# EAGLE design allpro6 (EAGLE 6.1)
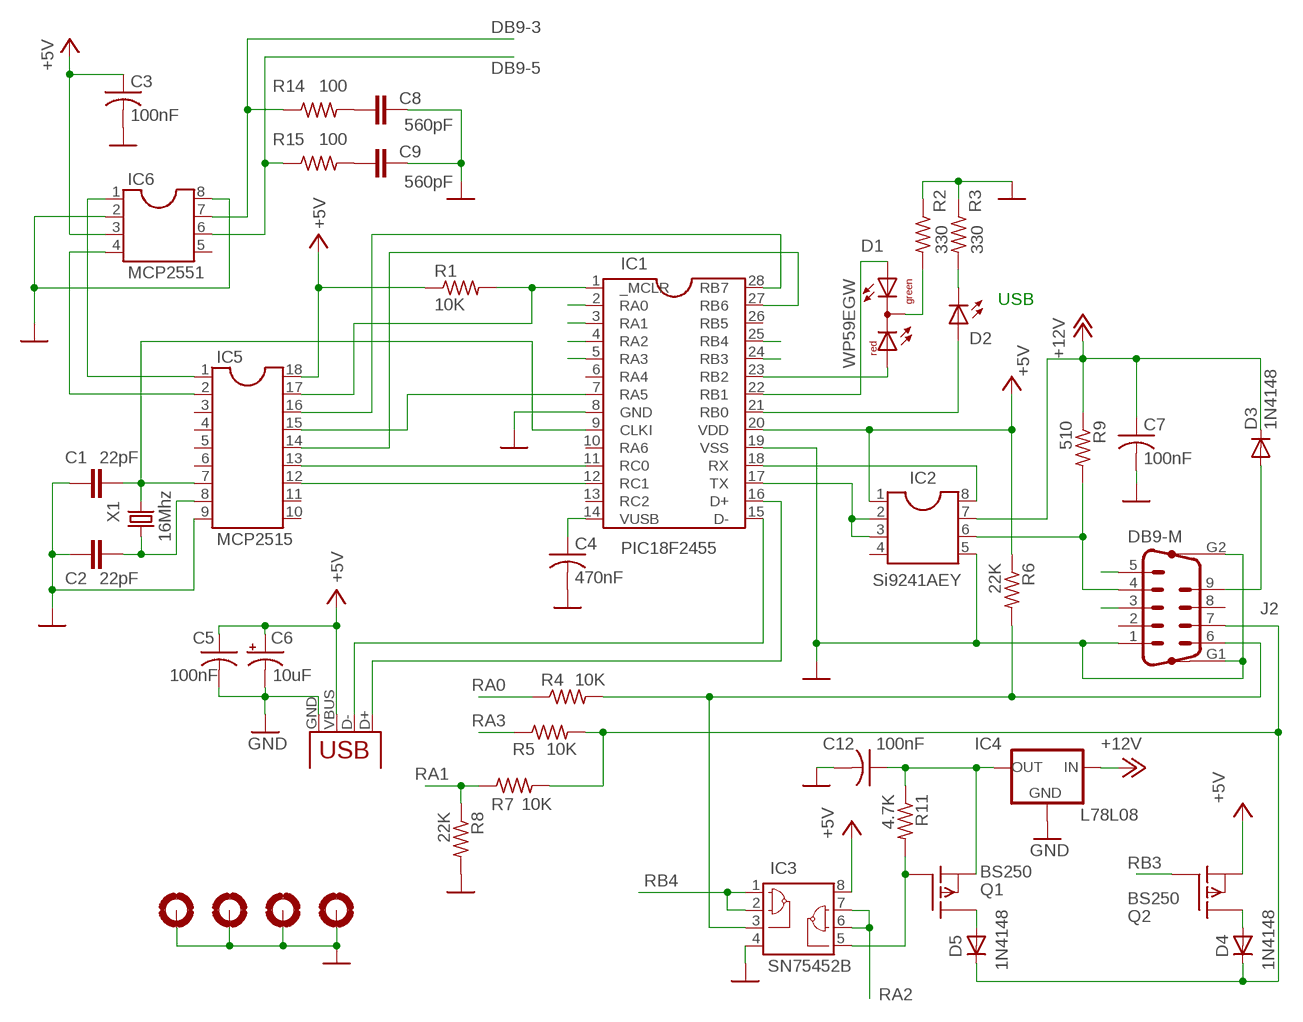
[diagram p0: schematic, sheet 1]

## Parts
C1  22pF  C2.5/2  [C2.5-2]
C2  22pF  C2.5/2  [C2.5-2]
C3  100nF  C-US050-025X075  [C050-025X075]
C4  470nF  C-US050-035X075  [C050-035X075]
C5  100nF  C-US050-025X075  [C050-025X075]
C6  10uF  CPOL-USE2-4  [E2-4]
C7  100nF  C-US050-025X075  [C050-025X075]
C8  560pF  C2.5/2  [C2.5-2]
C9  560pF  C2.5/2  [C2.5-2]
C12  100nF  C-US050-025X075  [C050-025X075]
D1  WP59EGW  DUOLED-RG-C  [DUOLED-C-5MM]
D2  LED5MM  [LED5MM]
D3  1N4148  1N4148M  [D035-10M]
D4  1N4148  1N4148M  [D035-10M]
D5  1N4148  1N4148M  [D035-10M]
H1  MOUNT-PAD-ROUND2.8  [2,8-PAD]
H2  MOUNT-PAD-ROUND2.8  [2,8-PAD]
H3  MOUNT-PAD-ROUND2.8  [2,8-PAD]
H4  MOUNT-PAD-ROUND2.8  [2,8-PAD]
IC1  PIC18F2455  PIC18F2455-EC  [DIL28]
IC2  Si9241AEY  SO-8  [SO-8]
IC3  SN75452B  [DIL08]
IC4  L78L08  78LXX  [78LXX]
IC5  MCP2515  DIL18  [DIL18]
IC6  MCP2551  DIL8  [DIL08]
J1  USB-B-H  [USB-B-H]
J2  DB9-M  M09HP  [M09HP]
Q1  BS250  [TO92]
Q2  BS250  [TO92]
R1  10K  R-US_0207/10  [0207/10]
R2  330  R-US_0207/10  [0207/10]
R3  330  R-US_0207/10  [0207/10]
R4  10K  R-US_0207/10  [0207/10]
R5  10K  R-US_0207/10  [0207/10]
R6  22K  R-US_0207/10  [0207/10]
R7  10K  R-US_0207/10  [0207/10]
R8  22K  R-US_0207/10  [0207/10]
R9  510  R-US_0207/10  [0207/10]
R11  4.7K  R-US_0207/10  [0207/10]
R14  100  R-US_0207/10  [0207/10]
R15  100  R-US_0207/10  [0207/10]
X1  16Mhz  CRYTALHC49S  [HC49/S]

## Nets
+5V: C3.1 C5.1 C6.+ IC1.20(VDD) IC2.1 IC3.8 IC5.18 IC6.3 J1.VBUS Q2.1(S) R1.1 R6.1
+12V: C7.1 D3.C IC2.7 IC4.IN R9.1
DB9-3: IC6.7 J2.3 R14.1
DB9-5: IC6.6 J2.5 R15.1
GND: C1.1 C2.2 C3.2 C4.2 C5.2 C6.- C7.2 C8.1 C9.1 C12.2 H1.B2,8(MOUNT) H2.B2,8(MOUNT) H3.B2,8(MOUNT) H4.B2,8(MOUNT) IC1.8(GND) IC1.19(VSS) IC2.5 IC3.4 IC4.GND IC5.9 IC6.2 IC6.8 J1.GND J2.1 J2.G1 J2.G2 R2.1 R3.1 R8.2
N$1: IC3.3 J2.6 R4.2 R6.2
N$3: D1.AR IC1.23(RB2)
N$4: IC5.2 IC6.4
N$5: D2.A IC1.21(RB0)
N$6: IC2.6 J2.4 R9.2
N$7: D3.A J2.9
N$8: D1.C R2.2
N$10: D2.K(C) R3.2
N$11: IC1.15(D-) J1.D-
N$12: IC1.16(D+) J1.D+
N$14: D1.AX(AG) IC1.22(RB1)
N$15: IC1.27(RB6) IC5.14
N$16: IC1.28(RB7) IC5.16
N$17: IC1.1(_MCLR) IC5.17 R1.2
N$18: D4.C D5.C J2.7 R5.2 R7.2
N$19: IC5.1 IC6.1
N$21: IC1.17(TX) IC2.2 IC2.3
N$22: C4.1 IC1.14(VUSB)
N$23: IC1.18(RX) IC2.8
N$25: D4.A Q2.3(D)
N$28: IC3.5 Q1.2(G) R11.2
N$35: C9.2 R15.2
N$36: C8.2 R14.2
N$37: IC1.7(RA5) IC5.15
N$40: C1.2 IC1.9(CLKI) IC5.7 X1.2
N$41: C2.1 IC5.8 X1.1
N$43: D5.A Q1.3(D)
N$45: C12.1 IC4.OUT Q1.1(S) R11.1
RA0: IC1.2(RA0) R4.1
RA1: IC1.3(RA1) R7.1 R8.1
RA2: IC1.4(RA2) IC3.6 IC3.7
RA3: IC1.5(RA3) R5.1
RB3: IC1.24(RB3) Q2.2(G)
RB4: IC1.25(RB4) IC3.1 IC3.2
RC0: IC1.11(RC0) IC5.13
RC1: IC1.12(RC1) IC5.12
Unconnected: IC1.6(RA4) IC1.10(RA6) IC1.13(RC2) IC1.26(RB5) IC2.4 IC5.3 IC5.4 IC5.5 IC5.6 IC5.10 IC5.11 IC6.5 J2.2 J2.8

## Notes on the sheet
- USB

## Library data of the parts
C1 C2 C8 C9 = capacitor-wima:C: CAPACITOR
C3-C5 C7 C12 = rcl:C-US: CAPACITOR, American symbol
C6 = rcl:CPOL-US: POLARIZED CAPACITOR, American symbol
D1 = led:DUOLED-RG-C: DUO LED 2 colors (red/green), 5 mm, round, common Cathode www.ligitek.com or other producers.
D2 = led:LED: LED
D3-D5 = diode:1N4148: DIODE
H1-H4 = holes:MOUNT-PAD-ROUND: MOUNTING PAD, round
IC1 = pic18f2455:PIC18F2455-EC
IC2 = so-8:SO-8
IC3 = 7545x:SN75452B
IC4 = v-reg:78LXX: VOLTAGE REGULATOR
IC5 = ic-package:DIL18: Dual In Line
IC6 = ic-package:DIL8: Dual In Line / Socket
J1 = con-usb:USB: USB Connectors
J2 = con-subd:M09HP: SUB-D; OC_FARNELL: unknown; OC_NEWARK: unknown
Q1 Q2 = transistor-fet:BS250: P-Channel Enhancement MOSFET -20V; -2A; 2,0Ohm
R1-R9 R11 R14 R15 = rcl:R-US_: RESISTOR, American symbol
X1 = crystal:CRYTAL: CRYSTAL

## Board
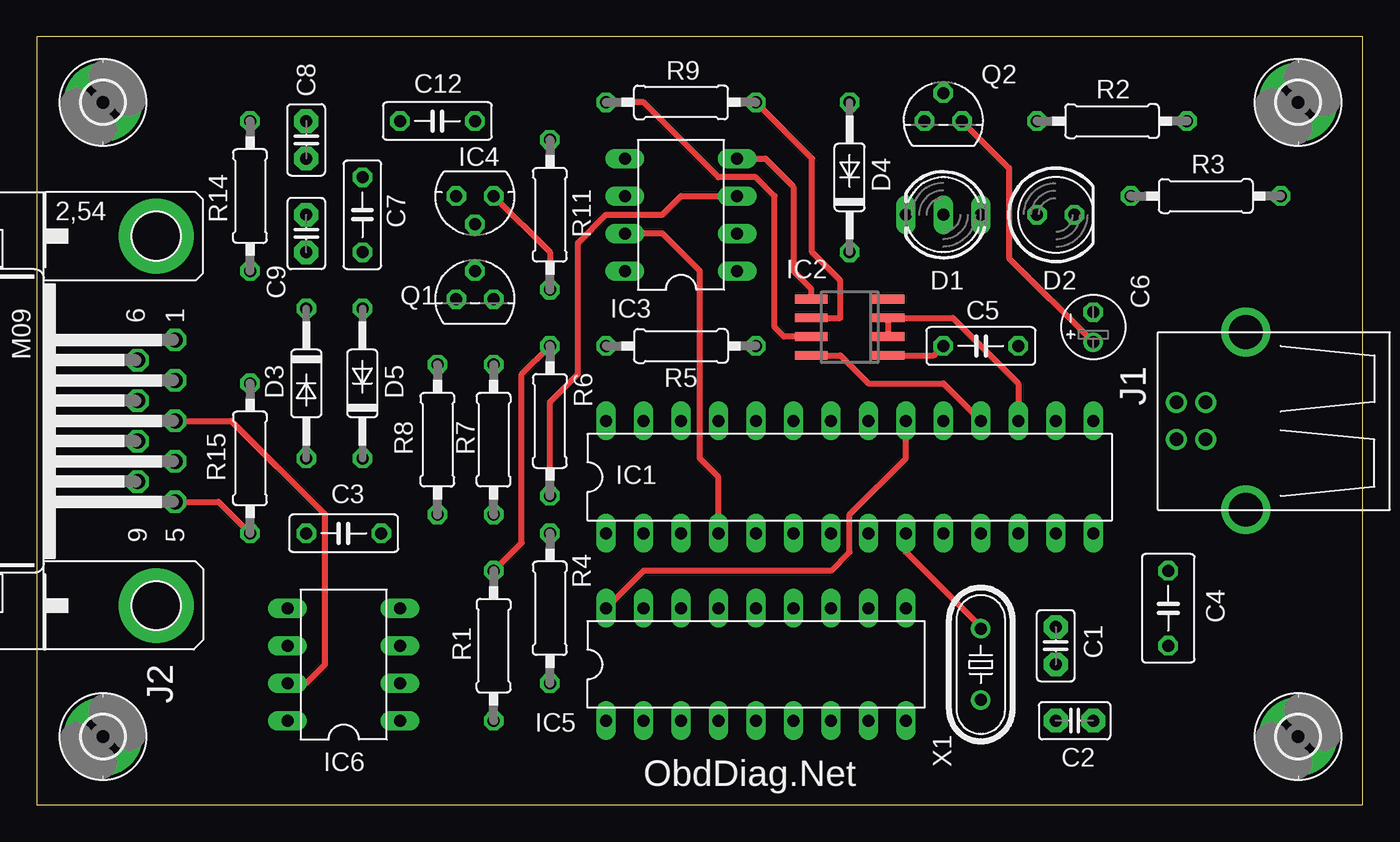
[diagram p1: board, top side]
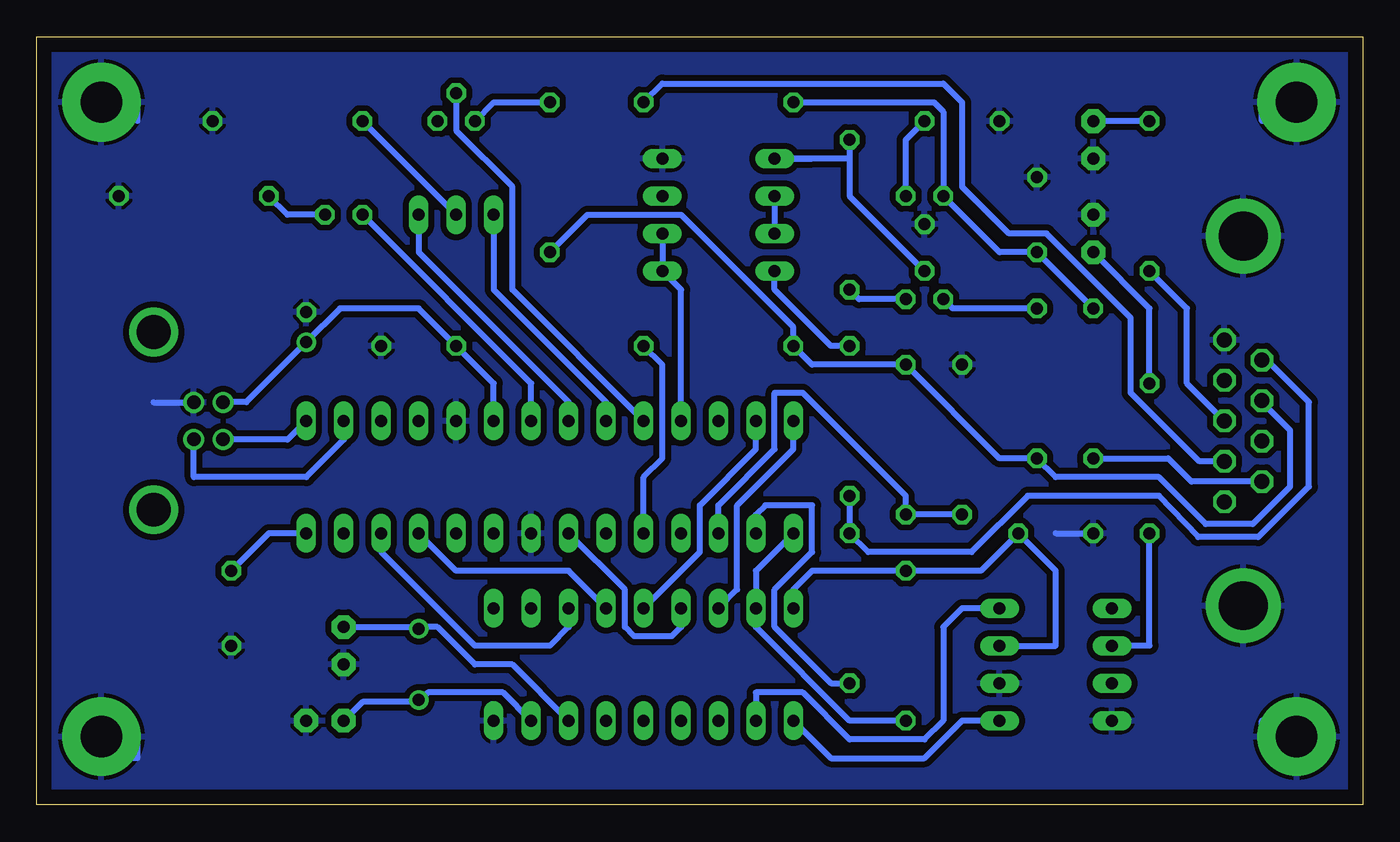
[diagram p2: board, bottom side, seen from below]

Size 89.84 x 52.06 mm. Coordinates in mm from the lower left corner, seen from the top.
Outline: 0,0 89.84,0 89.84,52.06 0,52.06 0,0
Copper layers (1*16): Top 0.035mm / dielectric 1.5mm / Bottom 0.035mm
Design rules: minimum track width 10mil, minimum drill 24mil, track to track 8mil, track to pad 8mil, pad to pad 8mil, via to via 8mil, smd to smd 8mil, copper to edge 40mil, drill to drill 8mil, minimum pad ring 10mil, minimum via ring 8mil, stop-mask expansion 4mil, vias tented up to drill 0mil, thermal gap 10mil

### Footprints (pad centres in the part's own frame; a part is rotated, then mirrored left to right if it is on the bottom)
C2.5-2 = drill 0.813 pad 1.6 octagon: 1 -1.27,0; 2 1.27,0
C050-025X075 = drill 0.813 octagon: 1 -2.54,0; 2 2.54,0
C050-035X075 = drill 0.813 octagon: 1 -2.54,0; 2 2.54,0
E2-4 = drill 0.813 pad 1.27: + -1.016,0 | drill 0.813 pad 1.27 octagon: - 1.016,0
DUOLED-C-5MM = drill 0.813 long: AR 2.54,0; AX -2.54,0; C 0,0
LED5MM = drill 0.813 octagon: A -1.27,0; K 1.27,0
D035-10M = drill 0.813 octagon: A 5.08,0; C -5.08,0
2,8-PAD = drill 2.8 pad 5.334: B2,8 0,0
DIL28 = drill 0.813 long: 1 -16.51,-3.81; 2 -13.97,-3.81; 3 -11.43,-3.81; 4 -8.89,-3.81; 5 -6.35,-3.81; 6 -3.81,-3.81; 7 -1.27,-3.81; 8 1.27,-3.81; 9 3.81,-3.81; 10 6.35,-3.81; 11 8.89,-3.81; 12 11.43,-3.81; 13 13.97,-3.81; 14 16.51,-3.81; 15 16.51,3.81; 16 13.97,3.81; 17 11.43,3.81; 18 8.89,3.81; 19 6.35,3.81; 20 3.81,3.81; 21 1.27,3.81; 22 -1.27,3.81; 23 -3.81,3.81; 24 -6.35,3.81; 25 -8.89,3.81; 26 -11.43,3.81; 27 -13.97,3.81; 28 -16.51,3.81
SO-8 = smd 0.6 x 2.2: 1 -1.905,-2.6; 2 -0.635,-2.6; 3 0.635,-2.6; 4 1.905,-2.6; 5 1.905,2.6; 6 0.635,2.6; 7 -0.635,2.6; 8 -1.905,2.6
DIL08 = drill 0.813 long: 1 -3.81,-3.81; 2 -1.27,-3.81; 3 1.27,-3.81; 4 3.81,-3.81; 5 3.81,3.81; 6 1.27,3.81; 7 -1.27,3.81; 8 -3.81,3.81
78LXX = drill 0.813 octagon: GND 0,1.905; IN 1.27,0; OUT -1.27,0
DIL18 = drill 0.813 long: 1 -10.16,-3.81; 2 -7.62,-3.81; 3 -5.08,-3.81; 4 -2.54,-3.81; 5 0,-3.81; 6 2.54,-3.81; 7 5.08,-3.81; 8 7.62,-3.81; 9 10.16,-3.81; 10 10.16,3.81; 11 7.62,3.81; 12 5.08,3.81; 13 2.54,3.81; 14 0,3.81; 15 -2.54,3.81; 16 -5.08,3.81; 17 -7.62,3.81; 18 -10.16,3.81
USB-B-H = drill 0.914: D+ 0,1.25; D- 1.981,1.25; GND 0,-1.25; VBUS 1.981,-1.25 | drill 2.286: P$1 -2.718,-6.02; P$2 -2.718,6.02
M09HP = drill 1.016 octagon: 1 -5.486,1.27; 2 -2.743,1.27; 3 0,1.27; 4 2.743,1.27; 5 5.486,1.27; 6 -4.115,-1.27; 7 -1.372,-1.27; 8 1.372,-1.27; 9 4.115,-1.27 | drill 3.302 pad 5.08: G1 -12.522,0; G2 12.522,0
TO92 = drill 0.813 octagon: 1 1.27,0; 2 0,1.905; 3 -1.27,0
0207/10 = drill 0.813 octagon: 1 -5.08,0; 2 5.08,0
HC49/S = drill 0.813: 1 -2.413,0; 2 2.413,0

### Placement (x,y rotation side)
C1  69.05,10.79 90 top
C2  70.32,5.71 0 top
C3  20.79,18.41 180 top
C4  76.67,13.33 270 top
C5  63.97,31.11 0 top
C6  71.59,32.38 90 top
C7  22.06,40 90 top
C8  18.25,45.08 90 top
C9  18.25,38.73 270 top
C12  27.14,46.35 180 top
D1  61.43,40 180 top
D2  69.05,40 0 top
D3  18.25,28.57 270 top
D4  55.08,42.54 90 top
D5  22.06,28.57 90 top
H1  4.47,4.63 0 top
H2  4.47,47.63 0 top
H3  85.47,4.63 0 top
H4  85.47,47.63 0 top
IC1  55.08,22.22 0 top
IC2  55.08,32.38 90 top
IC3  43.65,40 90 top
IC4  29.68,41.27 180 top
IC5  48.73,9.52 0 top
IC6  20.79,9.52 90 top
J1  79.21,26.03 180 top
J2  8.09,26.03 270 top
Q1  29.68,34.29 0 top
Q2  61.43,46.35 0 top
R1  30.95,10.79 270 top
R2  72.86,46.35 180 top
R3  79.21,41.27 180 top
R4  34.76,13.33 90 top
R5  43.65,31.11 180 top
R6  34.76,26.03 270 top
R7  30.95,24.76 90 top
R8  27.14,24.76 90 top
R9  43.65,47.62 0 top
R11  34.76,40 90 top
R14  14.44,41.27 90 top
R15  14.44,23.49 90 top
X1  63.97,9.52 90 top

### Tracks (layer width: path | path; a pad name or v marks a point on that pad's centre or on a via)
+5V
  Top 0.406: IC2.1 60.8,30.47 C5.1 | R1.1 32.85,17.77 32.85,29.2 R6.1 | Q2.1 65.88,43.18 65.88,37.08 C6.+ | IC5.18 41.11,15.87 53.81,15.87 55.08,17.14 55.08,19.68 58.89,23.49 IC1.20
  Bottom 0.406: J1.VBUS 76.69,27.28 76.67,27.3 75.65,27.3 C6.+ 69.3,33.65 63.97,33.65 C5.1 58.89,28.57 IC1.20 | IC6.3 20.79,10.79 20.79,15.87 C3.1 25.87,15.87 R1.1 37.3,15.87 38.57,14.6 IC5.18 | R6.1 36.03,31.11 39.84,34.92 IC3.8
+12V
  Top 0.406: IC2.7 50.63,31.74 50,32.38 50,41.27 48.73,42.54 46.19,42.54 41.11,47.62 R9.1
  Bottom 0.406: D3.C C7.1 24.6,37.46 IC4.IN 28.41,46.98 29.04,47.62 R9.1
DB9-3
  Top 0.406: IC6.7 18.25,8.25 19.52,9.52 19.52,19.68 13.17,26.03 J2.3
  Bottom 0.406: J2.3 11.9,28.57 11.9,33.65 R14.1
DB9-5
  Top 0.406: J2.5 12.31,20.54 R15.1
  Bottom 0.406: R15.1 14.44,10.79 IC6.6
GND
  Top 0.406: IC3.4 49.37,43.81 51.27,41.91 51.27,36.19 52.48,34.98 IC2.5
  Bottom 0.406: 20.79,18.41 C3.2 | 81.94,27.28 J1.GND | 6.57,47.62 6.82,47.62 6.82,46.35 | 6.82,4.44 6.82,5.71 | 83.02,46.35 83.02,47.62 | 83.02,4.44 83.02,3.17 85.56,3.17
  pour Bottom (isolate 0.406): 0.47,51.43 89.37,51.43 89.37,0.63 0.47,0.63
N$1
  Top 0.406: R6.2 34.76,27.3 36.66,29.2 36.66,38.1 38.57,40 42.38,40 43.65,41.27 IC3.3
  Bottom 0.406: R6.2 R4.2 33.49,17.14 26.5,17.14 22.7,20.95 13.81,20.95 11.14,18.16 7.07,18.16 3.64,21.58 3.64,27.3 6.49,30.14 J2.6
N$3
  Bottom 0.406: IC1.23 51.27,27.3 58.89,34.92 D1.AR
N$4
  Bottom 0.406: IC5.2 41.11,7.62 37.94,7.62 34.76,4.44 29.68,4.44 28.41,5.71 28.41,12.06 27.14,13.33 IC6.4
N$5
  Bottom 0.406: IC1.21 56.35,28.57 D2.A
N$6
  Top 0.406: IC2.6 54.45,33.02 54.45,35.55 52.54,37.46 52.54,43.81 R9.2
  Bottom 0.406: J2.4 11.06,23.29 15.71,27.93 15.71,33.02 21.42,38.73 23.96,38.73 27.14,41.91 27.14,47.62 28.41,48.89 47.46,48.89 R9.2
N$7
  Bottom 0.406: D3.A 13.17,23.49 11.6,21.91 J2.9
N$8
  Bottom 0.406: D1.C R2.2
N$10
  Bottom 0.406: D2.K 72.86,40 R3.2
N$11
  Bottom 0.406: IC1.15 72.86,24.76 77.21,24.76 J1.D-
N$12
  Bottom 0.406: J1.D+ 79.21,22.22 71.59,22.22 69.05,24.76 IC1.16
N$14
  Bottom 0.406: IC1.22 53.81,27.3 63.97,37.46 D1.AX
N$15
  Bottom 0.406: IC1.27 41.11,24.12 44.92,20.31 44.92,17.14 IC5.14
N$16
  Bottom 0.406: IC1.28 38.57,24.12 42.38,20.31 42.38,14.6 IC5.16
N$17
  Bottom 0.406: R1.2 34.76,5.71 41.11,12.06 IC5.17 41.11,15.87 IC1.1
N$18
  Bottom 0.406: D4.C 52.54,40 46.19,40 38.57,32.38 R5.2 37.3,29.84 R7.2 24.6,23.49 D5.C 20.79,22.22 13.81,22.22 10.63,19.04 7.46,19.04 4.92,21.58 4.92,25.39 6.82,27.3 J2.7
N$19
  Bottom 0.406: IC6.1 27.14,5.71 29.68,3.17 36.03,3.17 IC5.1
N$21
  Top 0.406: IC2.2 IC2.3 62.06,33.02 66.51,28.57 IC1.17
N$22
  Bottom 0.406: C4.1 74.13,18.41 IC1.14
N$23
  Top 0.406: IC1.18 61.43,28.57 56.35,28.57 54.45,30.47 IC2.8
N$25
  Bottom 0.406: Q2.3 58.89,47.62 D4.A
N$28
  Bottom 0.406: 37.3,43.81 IC3.5 34.76,43.81 | Q1.2 34.76,41.27 34.76,43.81 | R11.2 34.76,43.81
N$35
  Bottom 0.406: C9.2 14.44,33.65 R15.2
N$36
  Bottom 0.406: R14.2 C8.2
N$37
  Bottom 0.406: IC1.7 50,14.6 50,12.06 49.37,11.43 46.82,11.43 46.19,12.06 IC5.15
N$40
  Top 0.406: IC1.9 58.89,17.14 63.97,12.06 X1.2
  Bottom 0.406: 64.1,12.06 X1.2 | IC5.7 57.62,9.52 60.16,9.52 62.7,12.06 63.97,12.06 64.1,12.06 | C1.2 64.1,12.06
N$41
  Bottom 0.406: 63.97,6.98 X1.1 | 63.97,6.98 67.78,6.98 C2.1 | IC5.8 58.25,7.62 63.34,7.62 63.97,6.98
N$43
  Bottom 0.406: D5.A 27.77,33.65 Q1.3
N$45
  Top 0.406: IC4.OUT 34.76,37.46 R11.1
  Bottom 0.406: IC4.OUT 30.95,45.08 C12.1 | Q1.1 34.12,34.29 R11.1
RA0
  Bottom 0.406: IC1.2 41.11,19.68 40.48,20.31 37.3,20.31 37.3,17.14 39.84,14.6 39.84,12.06 36.03,8.25 R4.1
RA1
  Bottom 0.406: R8.1 R7.1 30.95,20.95 37.94,27.93 39.84,27.93 39.84,24.12 43.65,20.31 IC1.3
RA2
  Top 0.406: IC1.4 46.19,22.22 44.92,23.49 44.92,36.19 42.38,38.73 IC3.7
  Bottom 0.406: IC3.6 IC3.7
RA3
  Bottom 0.406: IC1.5 48.73,22.22 47.46,23.49 47.46,29.84 R5.1
RB3
  Bottom 0.406: IC1.24 57.62,34.92 57.62,41.91 61.43,45.72 Q2.2
RB4
  Bottom 0.406: IC3.2 IC3.1 46.19,34.92 IC1.25
RC0
  Bottom 0.406: IC5.13 53.81,15.87 61.43,15.87 IC1.11
RC1
  Bottom 0.406: IC1.12 66.51,17.14 60.16,10.79 55.08,10.79 53.81,12.06 IC5.12

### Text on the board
tNames: ObdDiag.Net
